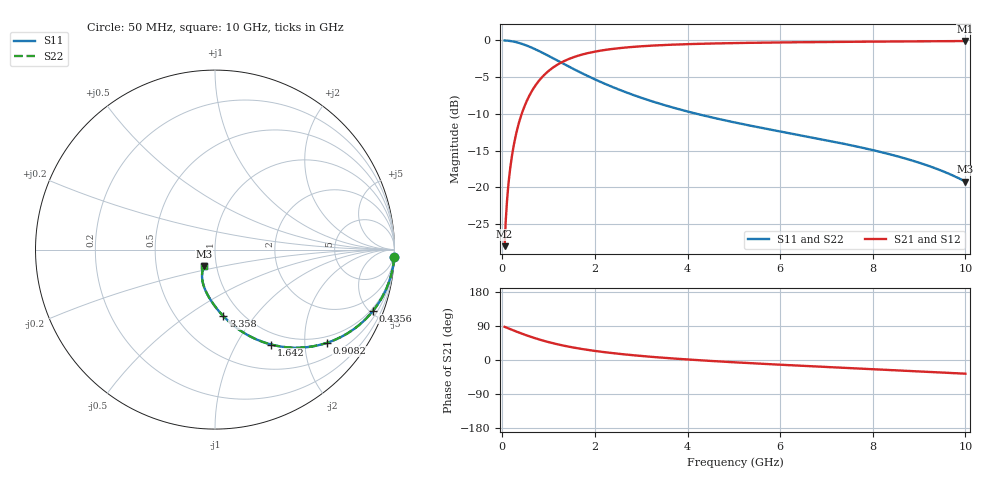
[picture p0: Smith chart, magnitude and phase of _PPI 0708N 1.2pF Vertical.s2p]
! S-Parameter data specifications (vertical orientation):
! Substrate: 40-mil Rogers 3003C, Substrate thickness, H=1.016mm, Dielectric constant, Er=3, Conductor thickness, T_mtl=0.043mm, Loss Tangent, Tand=0.003
! PCB Mounting Pad Footprint: Pad width, PadW=2.54mm , Pad length, PadL=0.51mm , Pad gap, PadG (edge-to-edge)=0.71mm , Reference planes=1.73mm apart
! Created Tue Jan 16 08:42:48 2018
# GHz S MA R 50
! 2 Port Network Data from SP1.SP block
! freq  magS11  angS11  magS21  angS21  magS12  angS12  magS22  angS22
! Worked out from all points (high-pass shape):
!   801 points, 50 MHz to 10 GHz, reference 50 ohm
!   highest |S21| = -0.09 dB at 10 GHz (marker M1); lowest = -28.0 dB at 50 MHz (marker M2)
!   |S21| within 3 dB of the highest: 1.251 GHz to end of sweep
!   lowest |S11| = -19.2 dB at 10 GHz (marker M3), VSWR 1.25, Z = 43.5 - j7.97 ohm
!   |S11| at or under -10 dB: 4.204 GHz to end of sweep
!   |S22| runs from -19.2 to 0.0 dB; largest |S21 - S12| = 0
!   S11 on the Smith chart (normalised r, x): 50 MHz: 1, -46; 435.6 MHz: 0.83, -5.25; 908.2 MHz: 0.83, -2.53; 1.642 GHz: 0.83, -1.41; 3.358 GHz: 0.82, -0.71; 10 GHz: 0.87, -0.16
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0.05  0.9992 -2.5  0.03977 87.5  0.03977 87.5  0.9992 -2.5
0.074875  0.9982 -3.7  0.0595 86.2  0.0595 86.2  0.9982 -3.7
0.1370625  0.9941 -6.8  0.1085 83.2  0.1085 83.2  0.9941 -6.8
0.19925  0.9876 -9.9  0.1566 80.1  0.1566 80.1  0.9876 -9.9
0.249  0.9809 -12.3  0.1943 77.7  0.1943 77.7  0.9809 -12.3
0.29875  0.9729 -14.7  0.2312 75.3  0.2312 75.3  0.9729 -14.7
0.4355625  0.9449 -21.1  0.3271 68.9  0.3271 68.9  0.9449 -21.1
0.647  0.8895 -30.1  0.4566 59.9  0.4566 59.9  0.8895 -30.1
0.9081875  0.812 -39.8  0.5832 50.2  0.5832 50.2  0.812 -39.8
1.219125  0.7213 -49.3  0.6919 40.7  0.6919 40.7  0.7213 -49.3
1.642  0.6152 -59.3  0.7875 30.6  0.7875 30.6  0.6152 -59.3
1.716625  0.5989 -60.8  0.7999 29.1  0.7999 29.1  0.5989 -60.8
2.052437  0.5338 -66.8  0.8446 23.1  0.8446 23.1  0.5338 -66.8
2.425562  0.4754 -72.3  0.8786 17.5  0.8786 17.5  0.4754 -72.3
3.358375  0.3743 -82.8  0.9259 7.0  0.9259 7.0  0.3743 -82.8
3.370812  0.3733 -82.9  0.9263 6.9  0.9263 6.9  0.3733 -82.9
4.117063  0.3212 -89.3  0.9454 0.5  0.9454 0.5  0.3212 -89.3
5.025  0.2762 -95.8  0.9592 -6.2  0.9592 -6.2  0.2762 -95.8
6.691625  0.2182 -106.1  0.9735 -16.6  0.9735 -16.6  0.2182 -106.1
8.345812  0.1686 -115.3  0.9827 -26.2  0.9827 -26.2  0.1686 -115.3
9.241312  0.1387 -120.2  0.9868 -31.5  0.9868 -31.5  0.1387 -120.2
10  0.1094 -124.2  0.99 -36.1  0.99 -36.1  0.1094 -124.2
